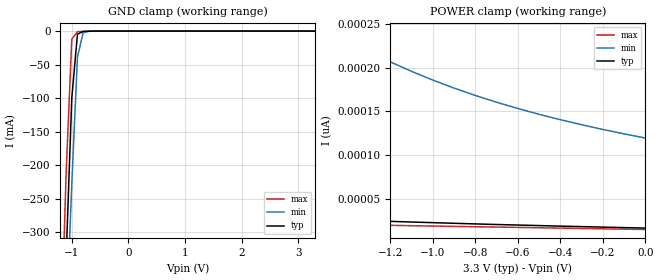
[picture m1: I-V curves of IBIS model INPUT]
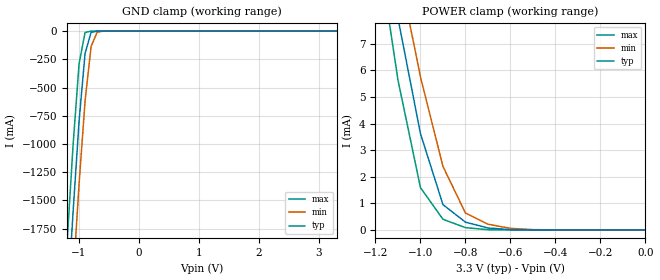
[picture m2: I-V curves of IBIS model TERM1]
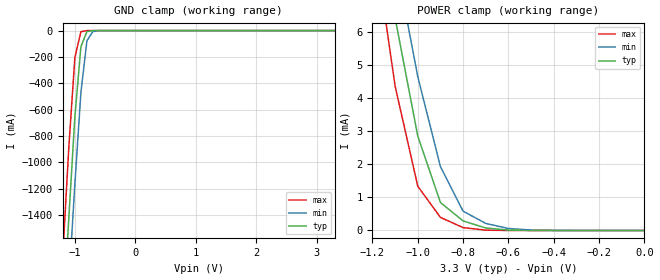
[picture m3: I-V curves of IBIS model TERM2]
|   PERICOM SEMICONDUCTOR CORP
|   IBIS Model of PI3A3899
|   Product Family: 3A
|   UQFN (ZT-16) Package
[IBIS Ver] 4.0
[Comment char] |_char
[File Name] pi3a3899_zt_33v.ibs
[File Rev] 1.0
[Source] File originated at Pericom Semiconductor Corp.
[Date] 04/10/18
[Disclaimer] (C) Copyright PERICOM Semiconductor Corporation
   All rights reserved
  Pericom Semiconductor Corporation hereby grants the user of
  this IBIS model a non-exclusive, nontransferable license to
  use this IBIS model under the following terms.
  This IBIS model is provided on an "AS IS" basis and Pericom
  makes absolutely no warranty with respect to the information
  contained herein. PERICOM DISCLAIMS AND CUSTOMER WAIVES ALL
  WARRANTIES, EXPRESSED OR IMPLIED, INCLUDING WARRANTIES OF
  MERCHANTABILITY OR FITNESS FOR A PARTICULAR PURPOSE. The
  entire risk as to quality and performance is with the customer.
  Accordingly, in no event shall the company be liable for any
  damages, whether in contract or tort, including any lost
  profits or other incidental, consequential, exemplary, or
  punitive damages arising out of the use or application of the
  IBIS model provided in this package. Further, Pericom reserves
  the right to make changes without notice to any product herein
  to improve reliability, function, or design. Pericom does not
  convey any license under patent rights or any other intellectual
  property rights, including those of third parties.
  The user is granted this license only to use the IBIS model
  and is not granted rights to sell, load, rent, lease or license
  the IBIS model in whole or in part, or in modified form to anyone
  other than user. User may modify the IBIS model to suit its specific
  application but rights to derivative works and such modifications
  shall belong to Pericom.
  Pericom is not obligated to provide maintenance or support
  for the licensed IBIS model.
  Contact Pericom at ATTN: APPLICATION ENGINEERING / IBIS MODELS
  2380 Bering Drive, San Jose, CA 95131
[Component] PI3A3899
[Manufacturer] Pericom Semiconductor Corp.
[Package]
| variable   typ   min   max
R_pkg   0.02106ohm   0.01714ohm   0.02498ohm
L_pkg   1.80200nH   1.61800nH   1.98600nH
C_pkg   0.10050pF   0.09950pF   0.10550pF
[Pin]  signal_name  model_name   R_pin   L_pin   C_pin
1   NC1   TERM2   0.02106   1.80200nH   0.10050pF
2   A0   INPUT   0.01714   1.61800nH   0.09950pF
3   NO2   TERM2   0.01714   1.61800nH   0.09950pF
4   COM2   TERM1   0.02106   1.80200nH   0.10050pF
5   NC2   TERM2   0.02498   1.98600nH   0.10550pF
6   GND   GND   0.02086   1.78900nH   0.10000pF
7   NO3   TERM2   0.02086   1.78900nH   0.10000pF
8   COM3   TERM1   0.02498   1.98600nh   0.10550pF
9   NC3   TERM2   0.02106   1.80200nH   0.10050pF
10   A1   INPUT   0.01714   1.61800nH   0.09950pF
11   NO4   TERM2   0.01714   1.61800nH   0.09950pF
12   COM4   TERM1   0.02106   1.80200nH   0.10050pF
13   NC4   TERM2   0.02498   1.98600nH   0.10550pF
14   VCC   POWER   0.02086   1.78900nH   0.10000pF
15   N01   TERM2   0.02086   1.78900nH   0.10000pF
16   COM1   TERM1   0.02498   1.98600nH   0.10550pF
[Series Switch Groups]
On 1 3 /
Off 2 4 /
[Series Pin Mapping]   pin_2   model_name  function_table_group
16   1   SWITCH1   1
4   5   SWITCH1   1
16   15   SWITCH1   2
4   3   SWITCH1   2
8   9   SWITCH1   3
12   13   SWITCH1   3
8   7   SWITCH1   4
12   11   SWITCH1   4
|   Model SWITCH1
[Model] SWITCH1
Model_type Series_switch
| variable   typ   min   max
C_comp   15.00pF   14.96pF   15.04pF
[Voltage Range]   3.3000V   3.0000V   3.6000V
[GND Clamp Reference]   0.0000V   0.0000V   0.0000V
[POWER Clamp Reference]   3.3000V   3.0000V   3.6000V
[Temperature Range]   25   85   -40
[On]
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[OFF]
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| Models and submodels in the file (4): INPUT (Input), SWITCH1 (Series_switch), TERM1 (Terminator), TERM2 (Terminator)
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|   Model INPUT
[Model] INPUT
Model_type Input
Vinl = 800mV
Vinh = 2.0V
| variable   typ   min   max
C_comp   1.650pF   1.640pF   1.660pF
[Voltage Range]   3.3000V   3.0000V   3.6000V
[GND Clamp Reference]   0.0000V   0.0000V   0.0000V
[POWER Clamp Reference]   3.3000V   3.0000V   3.6000V
[Temperature Range]   25   85   -40
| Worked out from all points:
|   GND clamp passes 1 mA (typ) near -0.81 V on its own axis
[GND Clamp]
| Voltage   I(typ)   I(min)   I(max)
-3.3V     -5.599A    -5.116A    -6.297A
-1.2V     -578.1mA   -653.2mA   -489mA
-1.1V     -339mA     -440.7mA   -212.4mA
-1V       -99.95mA   -228.2mA   -11.94mA
-900mV    -4.658mA   -38.85mA   -956.4uA
-800mV    -595.1uA   -2.415mA   -460.8uA
-700mV    -232.9uA   -358.7uA   -165.5uA
3.3V      16.05pA    134.8pA    13.22pA
[POWER Clamp]   |Note: Vtable = Vcc - Voutput
| Voltage   I(typ)   I(min)   I(max)
-3.3V     59.08pA    912.2pA    27.74pA
-2.9V     47.95pA    667pA      26.09pA
-2.5V     39.61pA    491pA      24.44pA
-2.1V     33.26pA    366.3pA    22.84pA
-1.5V     26.42pA    246.4pA    20.4pA
-1.4V     25.53pA    232pA      20.01pA
-1.3V     24.65pA    219pA      19.63pA
-1.1V     23.02pA    196pA      18.8pA
-800mV    20.85pA    168.4pA    17.61pA
-600mV    19.55pA    153.4pA    16.81pA
-400mV    18.3pA     140.6pA    16.02pA
0V        16.05pA    119.5pA    14.42pA
|   Model TERM1
[Model] TERM1
Model_type Terminator
| variable   typ   min   max
C_comp   7.000pF   6.980pF   7.020pF
[Voltage Range]   3.3000V   3.0000V   3.6000V
[GND Clamp Reference]   0.0000V   0.0000V   0.0000V
[POWER Clamp Reference]   3.3000V   3.0000V   3.6000V
[Temperature Range]   25   85   -40
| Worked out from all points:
|   GND clamp passes 1 mA (typ) near -0.71 V on its own axis
|   POWER clamp passes 1 mA (typ) near -0.90 V on its own axis
[GND Clamp]
| Voltage   I(typ)   I(min)   I(max)
-3.3V     -20.98A    -21.14A    -20.84A
-1.2V     -2.477A    -3.055A    -1.875A
-1.1V     -1.603A    -2.194A    -1.012A
-1V       -798.2mA   -1.355A    -289.5mA
-900mV    -196.9mA   -617.8mA   -12.67mA
-800mV    -12.36mA   -136.6mA   -127.8uA
-700mV    -335uA     -11.36mA   -974.9nA
-500mV    -159.8nA   -23.97uA   -396pA
3.3V      135.5pA    98.98nA    114.2pA
[POWER Clamp]   |Note: Vtable = Vcc - Voutput
| Voltage   I(typ)   I(min)   I(max)
-3.3V     3.569A     3.646A     3.507A
-1.2V     13.04mA    14.61mA    11.26mA
-1.1V     7.957mA    9.938mA    5.635mA
-1V       3.62mA     5.75mA     1.59mA
-900mV    951.2uA    2.387mA    402uA
-800mV    293.3uA    635uA      86.88uA
-700mV    75.4uA     216.5uA    9.89uA
-600mV    11.68uA    60.79uA    573.5nA
-500mV    951.1nA    13.21uA    17.55nA
0V        136.8pA    144.6pA    145.4pA
|   Model TERM2
[Model] TERM2
Model_type Terminator
| variable   typ   min   max
C_comp   7.000pF   6.980pF   7.020pF
[Voltage Range]   3.3000V   3.0000V   3.6000V
[GND Clamp Reference]   0.0000V   0.0000V   0.0000V
[POWER Clamp Reference]   3.3000V   3.0000V   3.6000V
[Temperature Range]   25   85   -40
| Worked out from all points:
|   GND clamp passes 1 mA (typ) near -0.71 V on its own axis
|   POWER clamp passes 1 mA (typ) near -0.91 V on its own axis
[GND Clamp]
| Voltage   I(typ)   I(min)   I(max)
-3.3V     -18.72A    -18.54A    -18.99A
-1.2V     -2.208A    -2.676A    -1.706A
-1.1V     -1.422A    -1.921A    -885.3mA
-1V       -654.5mA   -1.166A    -205.4mA
-900mV    -122.1mA   -468.6mA   -8.236mA
-800mV    -7.546mA   -76.09mA   -125.8uA
-700mV    -315.3uA   -6.468mA   -974.7nA
-500mV    -159.7nA   -23.3uA    -395.8pA
3.3V      83.69pA    98.92nA    67.01pA
[POWER Clamp]   |Note: Vtable = Vcc - Voutput
| Voltage   I(typ)   I(min)   I(max)
-3.3V     2.464A     2.484A     2.463A
-1.2V     10.87mA    12.4mA     9.119mA
-1.1V     6.419mA    8.242mA    4.357mA
-1V       2.851mA    4.644mA    1.335mA
-900mV    844.5uA    1.927mA    395uA
-800mV    288.5uA    582.4uA    86.32uA
-700mV    74.83uA    212.8uA    9.883uA
-600mV    11.66uA    60.24uA    573.3nA
-400mV    49.69nA    1.529uA    568.3pA
0V        83.81pA    137.2pA    90pA
